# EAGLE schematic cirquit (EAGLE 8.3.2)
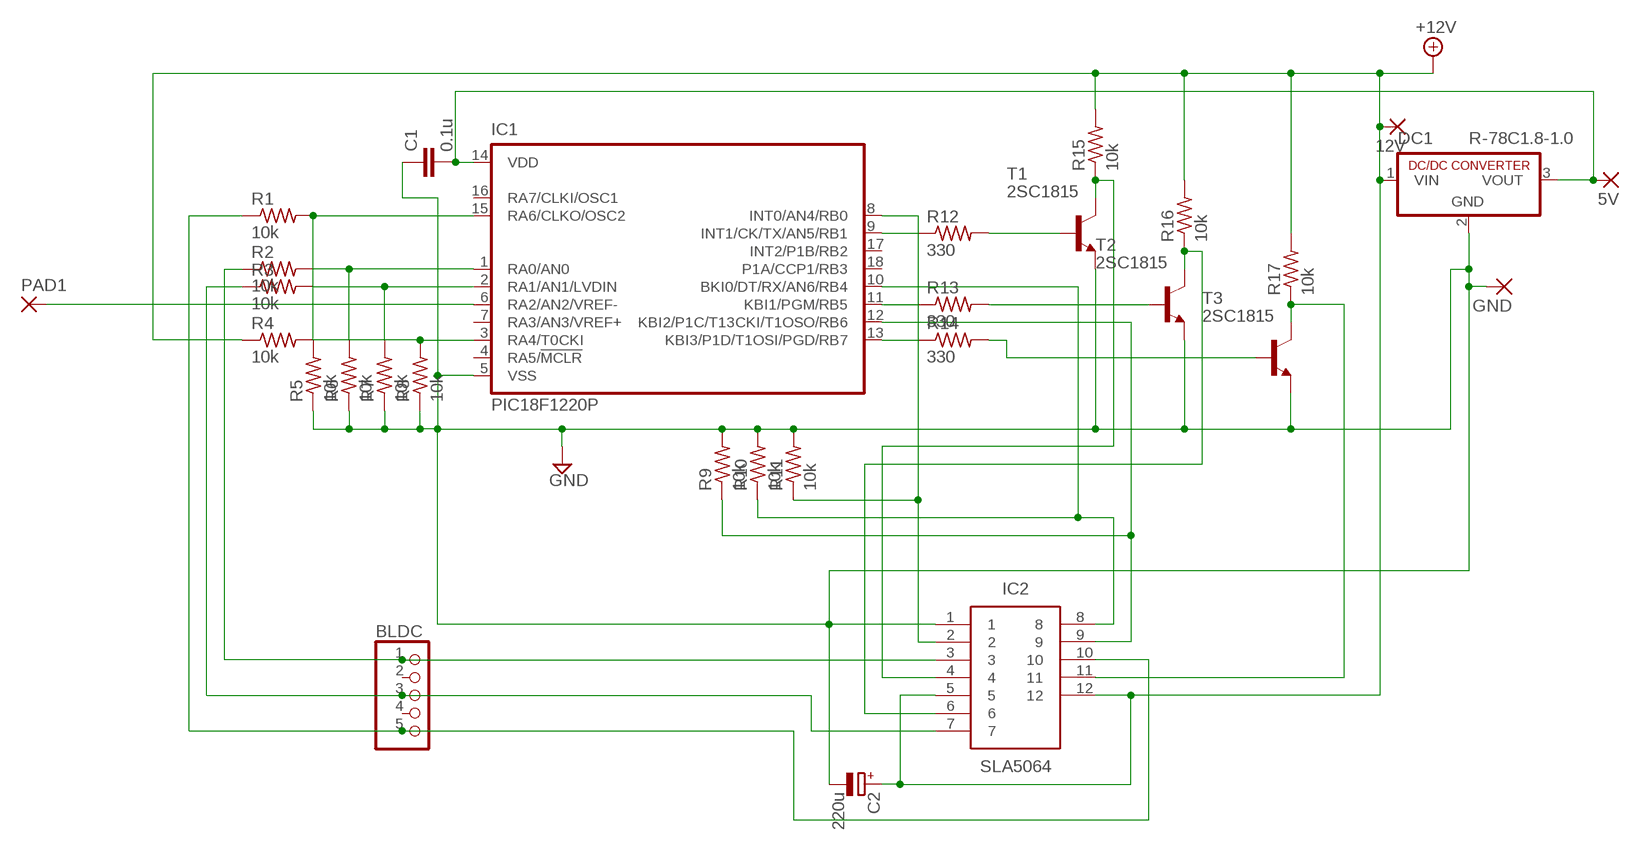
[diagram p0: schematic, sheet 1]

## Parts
5V  1,6/0,8  [1,6/0,8]
12V  1,6/0,8  [1,6/0,8]
BLDC  PINHD-1X5  [1X05]
C1  0.1u  C2.5/2  [C2.5-2]
C2  220u  CPOL-EUE2,5-6E  [E2,5-6E]
DC1  R-78C1.8-1.0  [SIP3]
GND  1,6/0,8  [1,6/0,8]
IC1  PIC18F1220P  [DIL18]
IC2  SLA5064  [TO254P500X3150X1890-12P]
PAD1  1,6/0,8  [1,6/0,8]
R1  10k  R-US_0204/7  [0204/7]
R2  10k  R-US_0204/7  [0204/7]
R3  10k  R-US_0204/7  [0204/7]
R4  10k  R-US_0204/7  [0204/7]
R5  10k  R-US_0204/7  [0204/7]
R6  10k  R-US_0204/7  [0204/7]
R7  10k  R-US_0204/7  [0204/7]
R8  10k  R-US_0204/7  [0204/7]
R9  10k  R-US_0204/7  [0204/7]
R10  10k  R-US_0204/7  [0204/7]
R11  10k  R-US_0204/7  [0204/7]
R12  330  R-US_0204/7  [0204/7]
R13  330  R-US_0204/7  [0204/7]
R14  330  R-US_0204/7  [0204/7]
R15  10k  R-US_0204/7  [0204/7]
R16  10k  R-US_0204/7  [0204/7]
R17  10k  R-US_0204/7  [0204/7]
T1  2SC1815  [TO92-ECB]
T2  2SC1815  [TO92-ECB]
T3  2SC1815  [TO92-ECB]

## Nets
+12V [power]: 12V.1(P) C2.+ DC1.1(VIN) IC2.5 IC2.12 R4.1 R15.2 R16.2 R17.2
GND [GND]: C1.1 C2.- DC1.2(GND) GND.1(P) IC1.5(VSS) IC2.1 R5.1 R6.1 R7.1 R8.1 R9.2 R10.2 R11.2 T1.E T2.E T3.E
N$1: IC1.15(RA6/CLKO/OSC2) R1.2 R5.2
N$2: IC1.1(RA0/AN0) R2.2 R6.2
N$3: IC1.2(RA1/AN1/LVDIN) R3.2 R7.2
N$4: IC1.3(RA4/T0CKI) R4.2 R8.2
N$6: BLDC.1 IC2.3 R2.1
N$7: BLDC.3 IC2.7 R3.1
N$9: IC1.9(INT1/CK/TX/AN5/RB1) R12.1
N$10: IC1.11(KBI1/PGM/RB5) R13.1
N$11: IC1.13(KBI3/P1D/T1OSI/PGD/RB7) R14.1
N$12: R12.2 T1.B
N$13: R13.2 T2.B
N$14: R14.2 T3.B
N$15: IC2.4 R15.1 T1.C
N$16: IC2.6 R16.1 T2.C
N$17: IC2.11 R17.1 T3.C
N$22: IC1.8(INT0/AN4/RB0) IC2.2 R11.1
N$23: IC1.10(BKI0/DT/RX/AN6/RB4) IC2.8 R10.1
N$24: IC1.12(KBI2/P1C/T13CKI/T1OSO/RB6) IC2.9 R9.1
N$25: IC1.6(RA2/AN2/VREF-) PAD1.1(P)
N$26: 5V.1(P) C1.2 DC1.3(VOUT) IC1.14(VDD)
N$29 [power]: BLDC.5 IC2.10 R1.1
Unconnected: BLDC.2 BLDC.4 IC1.4(RA5/!MCLR) IC1.7(RA3/AN3/VREF+) IC1.16(RA7/CLKI/OSC1) IC1.17(INT2/P1B/RB2) IC1.18(P1A/CCP1/RB3)

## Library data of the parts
5V 12V GND PAD1 = wirepad:1,6/0,8: THROUGH-HOLE PAD
BLDC = pinhead:PINHD-1X5: PIN HEADER
C1 = capacitor-wima:C: CAPACITOR
C2 = resistor:CPOL-EU: POLARIZED CAPACITOR, European symbol
DC1 = dc-dc-converter:R-78C*-1.0: INNOLINE DC/DC-Converter 1.0 AMP SIP3 Single Output Source: Data sheet
IC1 = microchip:PIC18F1*20: 18/20/28-Pin High-Performance, Enhanced Flash Microcontrollers with 10-bit A/D and nanoWatt Technology Source: ww1.microchip.com/downloads/en/DeviceDoc/39605c.pdf; MF: MICROCHIP; MPN: PIC18F1220-I/P; OC_FARNELL: 9761977; OC_NEWARK: 92C2429
IC2 = SLA5064:SLA5064: N-channel+P-channel 3-phase motor drive Source: Datasheet; DESCRIPTION: N-channel+P-channel 3-phase motor drive; HEIGHT: 5mm; MANUFACTURER_NAME: Sanken; MANUFACTURER_PART_NUMBER: SLA5064; SUPPLIER_NAME: RS
R1-R17 = resistor:R-US_: RESISTOR, American symbol
T1-T3 = transistor:2SC1815: NPN EPITAXIAL TRANSISTOR Source: TOSHIBA .. 2SC1815 1.pdf

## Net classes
0 default: width 0.178 mm, drill 0.5 mm, clearance 0.152 mm
1 power: width 2 mm, drill 0.5 mm, clearance 0.152 mm
2 GND: width 2 mm, drill 0.5 mm, clearance 0.152 mm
